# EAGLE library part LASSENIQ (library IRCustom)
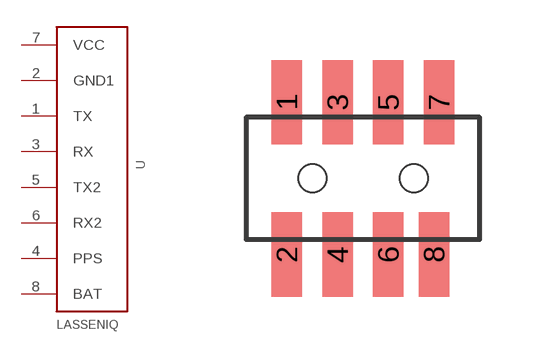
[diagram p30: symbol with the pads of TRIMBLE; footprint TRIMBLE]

Designator prefix -

## LASSENIQ  [TRIMBLE]
1  TX  out
2  GND1  sup
3  RX  in
4  PPS  out
5  TX2  out
6  RX2  in
7  VCC  sup
8  BAT  sup

## Footprint TRIMBLE (pad centres in mm)
smd 0.762 x 2.108: 1 -1.905,1.905; 2 -1.905,-1.905; 3 -0.635,1.905; 4 -0.635,-1.905; 5 0.635,1.905; 6 0.635,-1.905; 7 1.905,1.905; 8 1.778,-1.905
hole 0.7 at -1.27,0
hole 0.7 at 1.27,0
